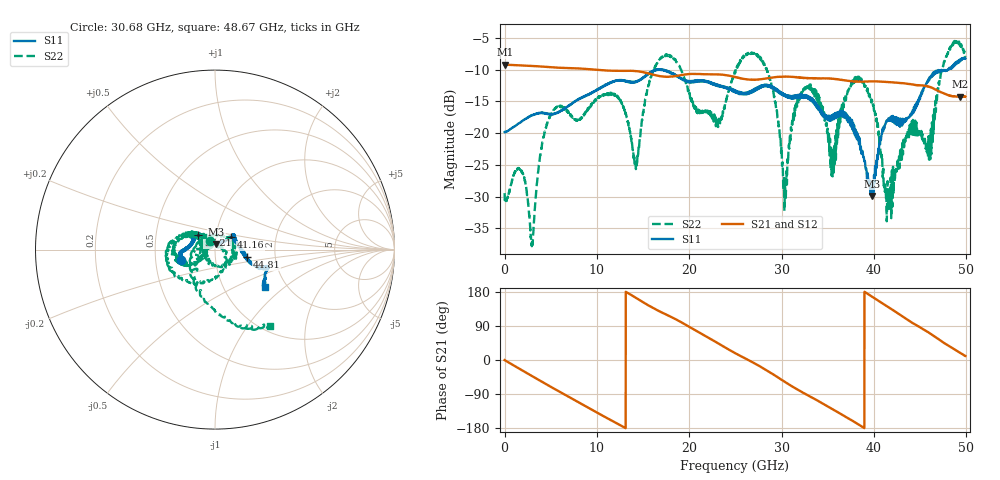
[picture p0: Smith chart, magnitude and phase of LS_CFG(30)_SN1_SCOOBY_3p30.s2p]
!Keysight Technologies,N5245B,MY58422026,A.13.80.08
!Date: Thursday, March 19, 2020 23:36:09
!Correction: S11(Full 2 Port(1,2))
!S21(Full 2 Port(1,2))
!S12(Full 2 Port(1,2))
!S22(Full 2 Port(1,2))
!S2P File: Measurements: S11, S21, S12, S22:
# Hz S DB R 50.0
!freq dBS11 angS11 dBS21 angS21 dBS12 angS12 dBS22 angS22
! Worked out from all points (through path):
!   4991 points, 10 MHz to 49.91 GHz, reference 50 ohm
!   highest |S21| = -9.21 dB at 20 MHz (marker M1); lowest = -14.3 dB at 49.35 GHz (marker M2)
!   group delay of S21, straight-line fit = 39 ps
!   lowest |S11| = -29.9 dB at 39.84 GHz (marker M3), VSWR 1.07, Z = 50.6 + j3.16 ohm
!   |S11| at or under -10 dB: start of sweep to 16.43 GHz; 16.46692 GHz to 16.53327 GHz (66.35 MHz wide, 0.402 % of centre); 17.07 GHz to 48.04 GHz (30.96 GHz wide, 95.1 % of centre)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
!   |S22| runs from -37.8 to -5.4 dB; largest |S21 - S12| = 0.0034
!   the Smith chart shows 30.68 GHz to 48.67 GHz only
!   S11 on the Smith chart (normalised r, x): 30.68 GHz: 0.68, -0.08; 37.21 GHz: 0.82, +0.13; 41.16 GHz: 1.18, +0.16; 44.81 GHz: 1.43, -0.13; 48.67 GHz: 1.57, -0.74
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1e7  -19.84 -2.0  -9.21 -0.3  -9.20 -0.3  -29.46 1.6
2e7  -19.87 -0.8  -9.21 -0.4  -9.20 -0.4  -30.23 -1.3
2.98e9  -17.16 -33.9  -9.43 -42.4  -9.42 -42.3  -37.41 -74.5
4.87e9  -16.99 -52.1  -9.61 -68.8  -9.60 -68.8  -17.56 -111.3
8.33e9  -14.49 -74.9  -9.85 -116.2  -9.84 -116.1  -17.59 -92.6
1.216e10  -11.76 -98.2  -10.20 -167.1  -10.19 -167.0  -14.17 -85.8
1.423e10  -11.97 -113.7  -10.23 164.0  -10.23 164.1  -25.68 -133.0
1.665e10  -10.01 -123.4  -10.98 130.1  -10.97 130.1  -8.69 -163.5
2.311e10  -12.59 -146.3  -10.74 44.4  -10.74 44.5  -18.75 -157.4
2.496e10  -13.42 -148.2  -11.15 18.3  -11.14 18.4  -10.47 -172.6
2.798e10  -12.52 -156.7  -11.48 -21.2  -11.47 -21.1  -8.68 -93.3
3.068e10  -14.21 -163.4  -11.10 -62.7  -11.10 -62.4  -24.88 118.6
3.328e10  -14.65 -178.8  -11.36 -99.1  -11.36 -98.7  -12.78 -167.5
3.553e10  -17.68 151.3  -11.42 -129.8  -11.36 -129.4  -26.82 -177.4
3.721e10  -18.27 139.3  -11.77 -153.8  -11.69 -153.9  -13.39 160.1
3.984e10  -29.92 77.9  -11.85 166.5  -11.83 166.5  -15.35 -96.6
4.116e10  -18.97 37.2  -11.92 145.8  -11.92 145.7  -28.04 17.4
4.16e10  -17.68 39.2  -11.97 139.0  -11.99 138.9  -28.79 109.4
4.481e10  -14.71 -13.6  -12.46 89.0  -12.47 89.1  -19.65 17.5
4.867e10  -9.13 -36.5  -14.24 28.9  -14.24 29.1  -5.62 -54.2
4.935e10  -8.48 -41.2  -14.29 18.6  -14.29 18.8  -5.76 -29.4
4.991e10  -8.25 -37.3  -14.25 10.5  -14.27 10.5  -7.85 -14.3
